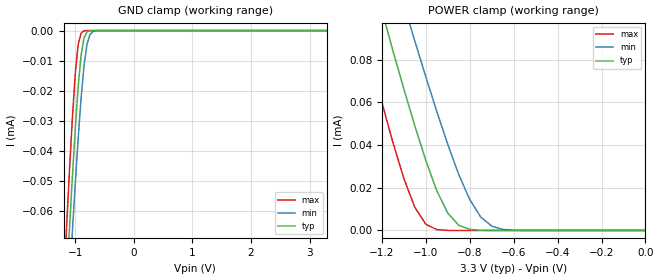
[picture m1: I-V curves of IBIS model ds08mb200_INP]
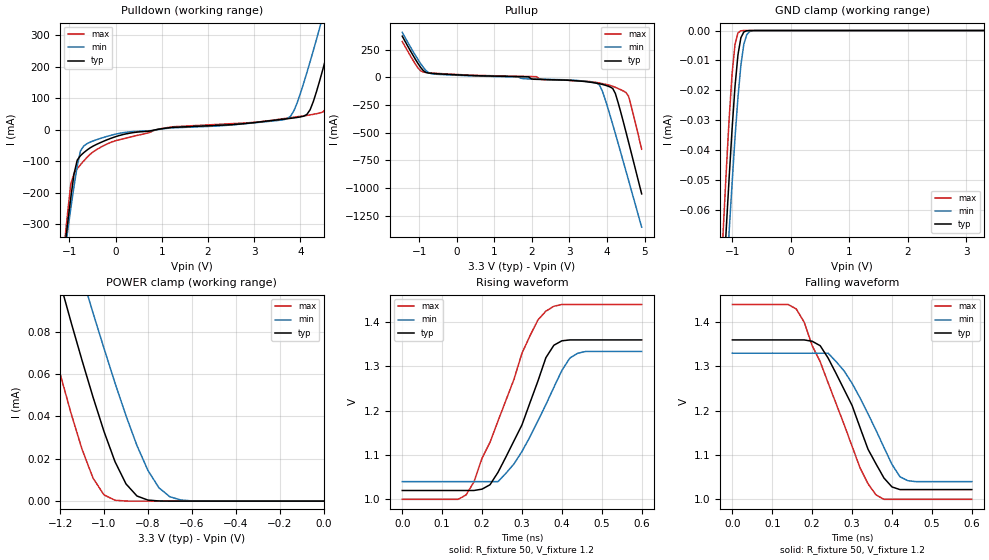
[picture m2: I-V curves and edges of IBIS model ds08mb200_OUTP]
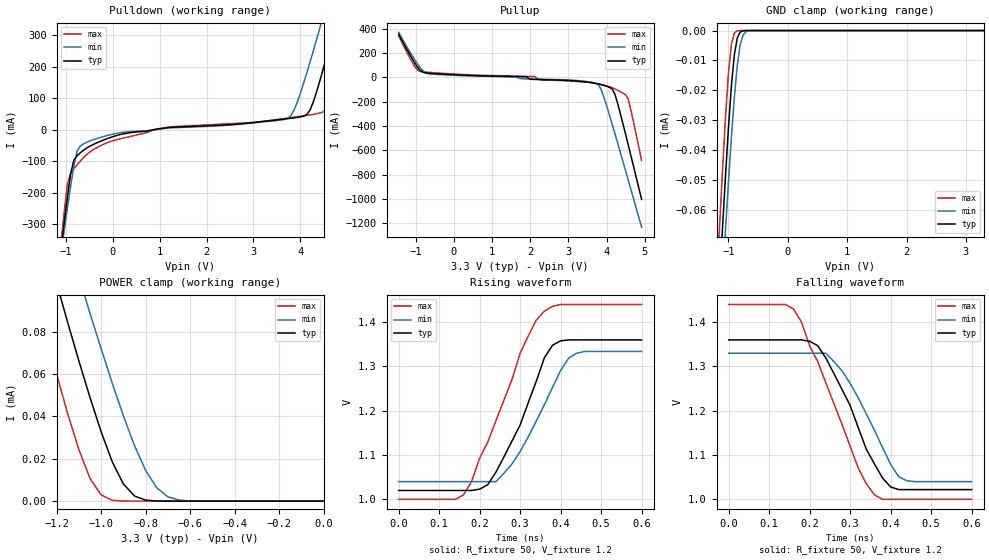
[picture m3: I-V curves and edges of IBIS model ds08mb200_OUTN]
|   National Semiconductor Corporation
|   IBIS Model
|   of
|   ds08mb200
|   Dual 0.8 Gbps 1:2/2:1 Mux Buffer
|   48 pin LLP package
[IBIS Ver]   3.2
[Comment Char]   |_char
[File name]   ds08mb200.ibs
[File Rev]   1.2
[Date]   01/30/06
[Source]
[Notes]
Created by Ivan Duzevik
Rev 1.0   The pre-emphasis (lvds_out)
   is not modeled due to the IBIS modeling limitations
   and design complexity.
Rev 1.1   Updated output models - dglisic
Rev 1.2   Added DS08MB200 pinout - lms
[Disclaimer]
(C) Copyright National Semiconductor Corporation 2005
   All rights reserved
   National Semiconductor Corporation hereby grants
the user of this IBIS model a non-exclusive, nontransferable
license to use this IBIS model under the following terms.
Before using this IBIS model, the user should read this
license.  If the user does not accept these terms,  the
IBIS model should be returned to National within 30 days.
   The user is granted this license only to use the
IBIS model and is not granted rights to sell, load, rent,
lease or license the IBIS model in whole or in part, or in
modified form to anyone other than user. User may modify
the IBIS model to suit its specific applications but rights
to derivative works and such modifications shall belong to
National.
   This IBIS model is provided on an "AS IS" basis and
National makes absolutely no warranty with respect to the
information contained herein.NATIONAL DISCLAIMS AND CUSTOMER
WAIVES ALL WARRANTIES, EXPRESS OR IMPLIED, INCLUDING
WARRANTIES OF MERCHANTABILITY OR FITNESS FOR A PARTICULAR
PURPOSE. The entire risk as to quality and performance is
with the Customer. ACCORDINGLY, IN NO EVENT SHALL THE
COMPANY BE LIABLE FOR ANY DAMAGES, WHETHER IN CONTRACT OR
TORT,INCLUDING ANY LOST PROFITS OR OTHER INCIDENTAL,
CONSEQUENTIAL, EXEMPLARY, OR PUNITIVE DAMAGES ARISING OUT
OF THE USE OR APPLICATION OF THE IBIS model provided in
this package.Further, National reserves the right to make
changes without notice to any product herein to improve
reliability, function, or design. National does not convey
any license under patent rights or any other intellectual
property rights, including those of third parties.
   National is not obligated to provide maintenance or support
for the licensed IBIS model.
Contact National at ATTN:INTERFACE/IBIS MODELS.
5 Foden Road, M/S 01-50, South Porltand, ME 04106
(207) 541-8609
[Copyright]
(c) Copyright 2005 National Semiconductor Corp.
[Component]   ds08mb200
Si_location Pin
Timing_location Pin
[Manufacturer]   National Semiconductor Corp.
[Package]
|   TYP   MIN   MAX
R_pkg   229m   215m   267m
L_pkg   1.4032n   1.2738n   1.6205n
C_pkg   0.0424p   0.0382p   0.0533p
[Pin]   signal_name   model_name   R_pin   L_pin   C_pin
1   NC   ds08mb200_CMOSIN   243m   1.4908n .0533p
2   GND   POWER   229m   1.4025n .0424p
3   GND   POWER   224m   1.3528n .0390p
4   EN_1   ds08mb200_CMOSIN   215m   1.3173n .0409p
5   NC   ds08mb200_CMOSIN   218m   1.3364n .0398p
6   VDD   POWER   232m   1.4032n .0393p
7   LO_1+   ds08mb200_OUTP   245m   1.4837n .0406p
8   LO_1-   ds08mb200_OUTN   267m   1.6205n .0523p
9   LI_1+   ds08mb200_INP   256m   1.5582n .0527p
10   LI_1-   ds08mb200_INN   236m   1.4593n .0415p
11   MUX_S1  ds08mb200_CMOSIN   231m   1.3840n .0408p
12   VDD   POWER   222m   1.3430n .0396p
13   ENA_1   ds08mb200_CMOSIN   212m   1.3258n .0408p
14   ENB_1   ds08mb200_CMOSIN   224m   1.2738n .0408p
15   SOA_1+  ds08mb200_OUTP   234m   1.4368n .0410p
16   SOA_1-  ds08mb200_OUTN   249m   1.5445n .0521p
17   SOB_1+  ds08mb200_OUTP   256m   1.5295n .0520p
18   SOB_1-  ds08mb200_OUTN   229m   1.3871n .0418p
19   SIA_1+  ds08mb200_INP   220m   1.3194n .0404p
20   SIA_1-  ds08mb200_INN   215m   1.2531n .0395p
21   SIB_1+  ds08mb200_INP   198m   1.2179n .0382p
22   SIB_1-  ds08mb200_INN   206m   1.2347n .0409p
23   NC   ds08mb200_CMOSIN   219m   1.3000n .0413p
24   NC   ds08mb200_CMOSIN   227m   1.3843n .0519p
25   NC   ds08mb200_CMOSIN   243m   1.4908n .0533p
26   NC   ds08mb200_CMOSIN   229m   1.4025n .0424p
27   SIB_0-  ds08mb200_INN   224m   1.3528n .0390p
28   SIB_0+  ds08mb200_INP   215m   1.3173n .0409p
29   SIA_0-  ds08mb200_INN   218m   1.3364n .0398p
30   SIA_0+  ds08mb200_INP   232m   1.4032n .0393p
31   SOB_0-  ds08mb200_OUTN   245m   1.4837n .0406p
32   SOB_0+  ds08mb200_OUTP   267m   1.6205n .0523p
33   SOA_0-  ds08mb200_OUTN   256m   1.5582n .0527p
34   SOA_0+  ds08mb200_OUTP   236m   1.4593n .0415p
35   ENB_0   ds08mb200_CMOSIN   231m   1.3840n .0408p
36   ENA_0   ds08mb200_CMOSIN   222m   1.3430n .0396p
37   VDD   POWER   212m   1.3258n .0408p
38   MUX_S0  ds08mb200_CMOSIN   224m   1.2738n .0408p
39   LI_0-   ds08mb200_INN   234m   1.4368n .0410p
40   LI_0+   ds08mb200_INP   249m   1.5445n .0521p
41   LO_0-   ds08mb200_OUTN   256m   1.5295n .0520p
42   LO_0+   ds08mb200_OUTP   229m   1.3871n .0418p
43   VDD   POWER   220m   1.3194n .0404p
44   PREL_0  ds08mb200_CMOSIN   215m   1.2531n .0395p
45   ENL_0   ds08mb200_CMOSIN   198m   1.2179n .0382p
46   GND   POWER   206m   1.2347n .0409p
47   GND   POWER   219m   1.3000n .0413p
48   VDD   POWER   227m   1.3843n .0519p
[Series Pin Mapping]   pin_2   model_name
9   10   term_resistor
19   20   term_resistor
21   22   term_resistor
28   27   term_resistor
30   29   term_resistor
40   39   term_resistor
[Diff Pin] inv_pin   vdiff   tdelay_typ   tdelay_min   tdelay_max
| The '+' pin is Diff_pin and the '-' pin is the inv_pin
| Receiver Vth = +/-100mV
7   8   0.05   0   0   0
9   10   0.05   0   0   0
15   16   0.05   0   0   0
17   18   0.05   0   0   0
19   20   0.05   0   0   0
21   22   0.05   0   0   0
28   27   0.05   0   0   0
30   29   0.05   0   0   0
32   31   0.05   0   0   0
34   33   0.05   0   0   0
40   39   0.05   0   0   0
42   41   0.05   0   0   0
|   Model resistor
[Model]   term_resistor
Model_type   Series
Polarity   Non-Inverting
C_comp   0.0pF   0.0pF   0.0pF
[Temperature Range] 25   85   -40
[Voltage Range]   3.300   3.0   3.6
| Resistance   ohm(typ)   ohm(min)   ohm(max)
[R Series]   100   85   115
| Models and submodels in the file (6): ds08mb200_INP (Input), ds08mb200_INN (Input), ds08mb200_OUTP (Output), ds08mb200_OUTN (Output), ds08mb200_CMOSIN (Input), term_resistor (Series)
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[Model]   ds08mb200_INP
Model_type Input
Vinh=0.05
Vinl=-0.05
C_comp   2pF   2pF   2pF
[Model Spec]
S_overshoot_high   3.3   3.0   3.6
S_overshoot_low   0.0   0.0   0.0
[Temperature Range]   25   85   -40
[Voltage Range]   3.3   3.0   3.6
[GND Clamp]
|V(groundclamp)   I(typ)   I(min)   I(max)
-3.3V     -945.7uA   -911.3uA   -990.7uA
-1.15V    -84.3uA    -101uA     -66uA
-1.1V     -66.3uA    -83.7uA    -47uA
-1.05V    -49uA      -67uA      -29.3uA
-1V       -32.8uA    -51uA      -14.4uA
-950mV    -18.6uA    -35.7uA    -4.63uA
-900mV    -8.13uA    -22.4uA    -803nA
-850mV    -2.42uA    -11.6uA    -85nA
-800mV    -493nA     -4.63uA    -7.57nA
-750mV    -80.3nA    -1.39uA    -657pA
-650mV    -1.78nA    -72.3nA    -4.9pA
3.3V      2.2fA      16fA       2.09fA
[POWER Clamp]
|Vtable   I(typ)   I(min)   I(max)
-3.3V     945.7uA    936uA      962.1uA
-1.3V     141uA      178uA      99.7uA
-1.2V     103uA      141uA      60uA
-1.15V    84.3uA     124uA      41.3uA
-1.1V     66.3uA     106uA      24.4uA
-1.05V    49uA       88.7uA     10.8uA
-1V       32.8uA     72uA       2.92uA
-900mV    8.13uA     40.3uA     40.3nA
-800mV    493nA      14.5uA     307pA
-750mV    80.3nA     6.3uA      26.5pA
-650mV    1.78nA     527nA      201fA
0V        2.2fA      2.73fA     2.22fA
[Model]   ds08mb200_OUTP
Model_type Output
Polarity Non-Inverting
Vref=1.2
Vmeas=1.2
Rref=50   | 100 Ohms Across Outputs OUTP and OUTM
Cref=0p
C_comp   3pF   3pF   3pF
[Temperature Range]   25   85   -40
[Voltage Range]   3.3   3.0   3.6
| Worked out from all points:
|   slope of the pulldown table from 0 to 0.495 V, typ, clamps not added: 33.1 ohm
|   slope of the pullup table from 0 to 0.495 V, typ, clamps not added: 68.2 ohm
|   rising waveform, R_fixture 50, V_fixture 1.2: 20-80 % time 94ps typ, 98.3ps min, 113ps max; typ from 1.02 V to 1.36 V
|   falling waveform, R_fixture 50, V_fixture 1.2: 20-80 % time 99ps typ, 97.1ps min, 115ps max; typ from 1.36 V to 1.02 V
[GND Clamp]
|V(groundclamp)   I(typ)   I(min)   I(max)
-3.3V     -945.7uA   -911.3uA   -990.7uA
-1.15V    -84.3uA    -101uA     -66uA
-1.1V     -66.3uA    -83.7uA    -47uA
-1.05V    -49uA      -67uA      -29.3uA
-1V       -32.8uA    -51uA      -14.4uA
-950mV    -18.6uA    -35.7uA    -4.63uA
-900mV    -8.13uA    -22.4uA    -803nA
-850mV    -2.42uA    -11.6uA    -85nA
-800mV    -493nA     -4.63uA    -7.57nA
-750mV    -80.3nA    -1.39uA    -657pA
-650mV    -1.78nA    -72.3nA    -4.9pA
3.3V      2.2fA      16fA       2.09fA
[POWER Clamp]
|Vtable   I(typ)   I(min)   I(max)
-3.3V     945.7uA    936uA      962.1uA
-1.3V     141uA      178uA      99.7uA
-1.2V     103uA      141uA      60uA
-1.15V    84.3uA     124uA      41.3uA
-1.1V     66.3uA     106uA      24.4uA
-1.05V    49uA       88.7uA     10.8uA
-1V       32.8uA     72uA       2.92uA
-900mV    8.13uA     40.3uA     40.3nA
-800mV    493nA      14.5uA     307pA
-750mV    80.3nA     6.3uA      26.5pA
-650mV    1.78nA     527nA      201fA
0V        2.2fA      2.73fA     2.22fA
[Pullup]
|Vtable   I(typ)   I(min)   I(max)
-1.45V    372mA      406.3mA    323.4mA
-960mV    88.99mA    123.2mA    58.38mA
-820mV    44.22mA    61.17mA    43.46mA
-680mV    35.49mA    32.86mA    39.05mA
2.12V     -18.68mA   -16.56mA   5.425mA
3.1V      -30.26mA   -26.07mA   -30.28mA
3.8V      -58.72mA   -70.62mA   -52.39mA
3.94V     -70.87mA   -190.4mA   -62.41mA
4.15V     -101.1mA   -426.5mA   -81.69mA
4.22V     -146.4mA   -509mA     -90.91mA
4.57V     -584.3mA   -930.1mA   -169.7mA
4.92V     -1.054A    -1.355A    -650.7mA
[Pulldown]
|V(pulldown)   I(typ)   I(min)   I(max)
-2.02V    -1.566A    -1.42A     -1.773A
-1.11V    -386.2mA   -400mA     -366.9mA
-1.04V    -299.3mA   -324.2mA   -266.2mA
-970mV    -216.2mA   -250.3mA   -173.1mA
-760mV    -82.25mA   -66.98mA   -111.1mA
-200mV    -32.82mA   -21.76mA   -46.22mA
3.65V     33.82mA    32.26mA    35.55mA
3.86V     37.56mA    60.38mA    39.89mA
4.14V     48.47mA    181.2mA    45.54mA
4.42V     156.9mA    324.9mA    53.13mA
4.7V      310.2mA    524.2mA    129.1mA
4.91V     432mA      725.1mA    251.3mA
[Rising Waveform]
R_fixture=50
V_fixture=1.2
V_fixture_min=1.2
V_fixture_max=1.2
0s        1.02V      1.04V      1V
160ps     1.02V      1.04V      1.01V
220ps     1.033V     1.04V      1.129V
240ps     1.061V     1.04V      1.177V
300ps     1.168V     1.108V     1.33V
340ps     1.267V     1.177V     1.405V
360ps     1.32V      1.214V     1.425V
400ps     1.358V     1.291V     1.44V
440ps     1.36V      1.33V      1.44V
600ps     1.36V      1.334V     1.44V
[Falling Waveform]
R_fixture=50
V_fixture=1.2
V_fixture_min=1.2
V_fixture_max=1.2
0s        1.36V      1.33V      1.44V
160ps     1.36V      1.33V      1.43V
220ps     1.347V     1.33V      1.311V
240ps     1.319V     1.33V      1.263V
280ps     1.248V     1.29V      1.169V
320ps     1.162V     1.229V     1.071V
360ps     1.08V      1.156V     1.01V
400ps     1.028V     1.079V     1V
420ps     1.022V     1.051V     1V
600ps     1.022V     1.04V      1V
[Ramp]
|   typ   min   max
dV/dt_r   205m/100p   175m/90p   242m/115p
dV/dt_f   205m/100p   175m/90p   242m/115p
R_load=50
|[End   ds08mb200_OUTP
[Model]   ds08mb200_OUTN
Model_type Output
Polarity Inverting
Vref=1.2
Vmeas=1.2
Rref=50   | 100 Ohms Across Outputs OUTP and OUTM
Cref=0p
C_comp   3pF   3pF   3pF
[Temperature Range]   25   85   -40
[Voltage Range]   3.3   3.0   3.6
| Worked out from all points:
|   slope of the pulldown table from 0 to 0.495 V, typ, clamps not added: 33.1 ohm
|   slope of the pullup table from 0 to 0.495 V, typ, clamps not added: 71.6 ohm
|   rising waveform, R_fixture 50, V_fixture 1.2: 20-80 % time 94ps typ, 98.3ps min, 113ps max; typ from 1.02 V to 1.36 V
|   falling waveform, R_fixture 50, V_fixture 1.2: 20-80 % time 99ps typ, 97.1ps min, 115ps max; typ from 1.36 V to 1.02 V
[GND Clamp]
|V(groundclamp)   I(typ)   I(min)   I(max)
-3.3V     -945.7uA   -911.3uA   -990.7uA
-1.15V    -84.3uA    -101uA     -66uA
-1.1V     -66.3uA    -83.7uA    -47uA
-1.05V    -49uA      -67uA      -29.3uA
-1V       -32.8uA    -51uA      -14.4uA
-950mV    -18.6uA    -35.7uA    -4.63uA
-900mV    -8.13uA    -22.4uA    -803nA
-850mV    -2.42uA    -11.6uA    -85nA
-800mV    -493nA     -4.63uA    -7.57nA
-750mV    -80.3nA    -1.39uA    -657pA
-650mV    -1.78nA    -72.3nA    -4.9pA
3.3V      2.2fA      16fA       2.09fA
[POWER Clamp]
|Vtable   I(typ)   I(min)   I(max)
-3.3V     945.7uA    936uA      962.1uA
-1.3V     141uA      178uA      99.7uA
-1.2V     103uA      141uA      60uA
-1.15V    84.3uA     124uA      41.3uA
-1.1V     66.3uA     106uA      24.4uA
-1.05V    49uA       88.7uA     10.8uA
-1V       32.8uA     72uA       2.92uA
-900mV    8.13uA     40.3uA     40.3nA
-800mV    493nA      14.5uA     307pA
-750mV    80.3nA     6.3uA      26.5pA
-650mV    1.78nA     527nA      201fA
0V        2.2fA      2.73fA     2.22fA
[Pullup]
|Vtable   I(typ)   I(min)   I(max)
-1.45V    354.3mA    369.4mA    340.4mA
-960mV    84.75mA    112mA      61.45mA
-680mV    33.8mA     29.87mA    41.1mA
2.12V     -17.79mA   -15.05mA   5.711mA
2.26V     -19.03mA   -16.11mA   -21.08mA
3.1V      -28.82mA   -23.7mA    -31.87mA
3.8V      -55.92mA   -64.2mA    -55.15mA
3.94V     -67.5mA    -173.1mA   -65.69mA
4.15V     -96.29mA   -387.7mA   -85.99mA
4.22V     -139.4mA   -462.7mA   -95.69mA
4.57V     -556.5mA   -845.5mA   -178.6mA
4.92V     -1.004A    -1.232A    -684.9mA
[Pulldown]
|V(pulldown)   I(typ)   I(min)   I(max)
-2.02V    -1.566A    -1.42A     -1.773A
-1.11V    -386.2mA   -400mA     -366.9mA
-1.04V    -299.3mA   -324.2mA   -266.2mA
-970mV    -216.2mA   -250.3mA   -173.1mA
-760mV    -82.25mA   -66.98mA   -111.1mA
-200mV    -32.82mA   -21.76mA   -46.22mA
3.65V     33.82mA    32.26mA    35.55mA
3.86V     37.56mA    60.38mA    39.89mA
4.14V     48.47mA    181.2mA    45.54mA
4.42V     156.9mA    324.9mA    53.13mA
4.7V      310.2mA    524.2mA    129.1mA
4.91V     432mA      725.1mA    251.3mA
[Rising Waveform]
R_fixture=50
V_fixture=1.2
V_fixture_min=1.2
V_fixture_max=1.2
0s        1.02V      1.04V      1V
160ps     1.02V      1.04V      1.01V
220ps     1.033V     1.04V      1.129V
240ps     1.061V     1.04V      1.177V
300ps     1.168V     1.108V     1.33V
340ps     1.267V     1.177V     1.405V
360ps     1.32V      1.214V     1.425V
400ps     1.358V     1.291V     1.44V
440ps     1.36V      1.33V      1.44V
600ps     1.36V      1.334V     1.44V
[Falling Waveform]
R_fixture=50
V_fixture=1.2
V_fixture_min=1.2
V_fixture_max=1.2
0s        1.36V      1.33V      1.44V
160ps     1.36V      1.33V      1.43V
220ps     1.347V     1.33V      1.311V
240ps     1.319V     1.33V      1.263V
280ps     1.248V     1.29V      1.169V
320ps     1.162V     1.229V     1.071V
360ps     1.08V      1.156V     1.01V
400ps     1.028V     1.079V     1V
420ps     1.022V     1.051V     1V
600ps     1.022V     1.04V      1V
[Ramp]
|   typ   min   max
dV/dt_r   205m/100p   175m/90p   242m/115p
dV/dt_f   205m/100p   175m/90p   242m/115p
R_load=50
|[End   ds08mb200_OUTN
